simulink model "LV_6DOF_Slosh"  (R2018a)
settings: Solver=FixedStepAuto  StartTime=0.0  StopTime=489.8  FixedStep=0.0002  MaxStep=0.0001  RelTol=2e-6  EnableMultiTasking=on
InitFcn:
  | init
StopFcn:
  | pl
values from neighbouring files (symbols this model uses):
  accel = [97.3083,0,0]    [init.m]
  AcNoise = 0.1    [init.m]
  BBrcs = [82, 0.0, +3.375]    [init.m]
  Cdelay = 0.005    [init.m]
  Cza1 = FCS_Gains_Stg1(:, 5)    [init.m]
  d2r = pi/180    (= 0.0174532925199)    [init.m]    (also in pl.m; LQR_Design.m)
  Euler_0 = [90, 89.98, 0]*d2r    [init.m]
  fairing_mass = 1047.7*kg2slug    (= 71.7904994)    [init.m]
  Ie1 = 28.17    [init.m]
  Ie2 = 258.74    [init.m]
  Islosh = 1    [init.m]
  Isp = 65    [init.m]
  Ixxpr = Mass_Props(:,2)    [init.m]
  Ixypr = Mass_Props(:,5)    [init.m]
  Ixzpr = Mass_Props(:,6)    [init.m]
  Iyypr = Mass_Props(:,3)    [init.m]
  Iyzpr = Mass_Props(:,7)    [init.m]
  Izzpr = Mass_Props(:,4)    [init.m]
  Jdir = zeros(3,nt)    [init.m]
  JJ1 = Commands_2(:,2)    [init.m]
  JJ2 = Commands_2(:,3)    [init.m]
  JJ3 = Commands_2(:,4)    [init.m]
  Jloc = Jdir    [init.m]
  K_estim1 = FCS_Gains_Stg1(:,21)    [init.m]
  Kl_p1 = FCS_Gains_Stg1(:,12)    [init.m]
  Kl_phi1 = FCS_Gains_Stg1(:,11)    [init.m]
  Km_alfa1 = FCS_Gains_Stg1(:, 8)    [init.m]
  Km_alfin = FCS_Gains_Stg1(:,10)    [init.m]
  Km_q1 = FCS_Gains_Stg1(:, 7)    [init.m]
  Km_q2 = FCS_Gains_Stg2(:,5)    [init.m]
  Km_thet1 = FCS_Gains_Stg1(:, 6)    [init.m]
  Km_thet2 = FCS_Gains_Stg2(:,4)    [init.m]
  Km_thin1 = FCS_Gains_Stg1(:, 9)    [init.m]
  Km_thin2 = FCS_Gains_Stg2(:,6)    [init.m]
  Kmix2 = [ 0,   -1,    0;          0,    0,   -1]    [init.m]
  Kml1_1 = ee*FCS_Gains_Stg1(:,18)    [init.m]
  Kml2_1 = ee*FCS_Gains_Stg1(:,19)    [init.m]
  Kml2_2 = ee*FCS_Gains_Stg2(:,10)    [init.m]
  Kn_beta1 = FCS_Gains_Stg1(:,15)    [init.m]
  Kn_betin = FCS_Gains_Stg1(:,17)    [init.m]
  Kn_psi1 = FCS_Gains_Stg1(:,13)    [init.m]
  Kn_psi2 = FCS_Gains_Stg2(:,7)    [init.m]
  Kn_psin1 = FCS_Gains_Stg1(:,16)    [init.m]
  Kn_psin2 = FCS_Gains_Stg2(:,9)    [init.m]
  Kn_r1 = FCS_Gains_Stg1(:,14)    [init.m]
  Kn_r2 = FCS_Gains_Stg2(:,8)    [init.m]
  Le1 = 1.203    [init.m]
  Le2 = 2.892    [init.m]
  Massgn1 = ee*FCS_Gains_Stg1(:,2)    [init.m]
  Massgn2 = ee*FCS_Gains_Stg2(:,2)    [init.m]
  mdot1 = 2.5058    [init.m]
  mdot2 = 2.5058    [init.m]
  me1 = 9.325    [init.m]
  me2 = 13.927    [init.m]
  mrc = [x_ref, y_ref, z_ref]    [init.m]
  Msfue = Slosh(:,3)    [init.m]
  Mslox = Slosh(:,2)    [init.m]
  msspr = Mass_Props(:,1)    [init.m]
  Mvsls = Slosh(:,1)    [init.m]
  post_sep_wait = 4    [init.m]
  pre_sep_wait = 4    [init.m]
  Qbar1 = FCS_Gains_Stg1(:, 4)    [init.m]
  qtc1 = interp1(timi2(1:iend),Commands_2(1:iend, 9),timi2,'linear','extrap')    [init.m]
  qtc2 = interp1(timi2(1:iend),Commands_2(1:iend,10),timi2,'linear','extrap')    [init.m]
  qtc3 = interp1(timi2(1:iend),Commands_2(1:iend,11),timi2,'linear','extrap')    [init.m]
  qtc4 = interp1(timi2(1:iend),Commands_2(1:iend,12),timi2,'linear','extrap')    [init.m]
  r2d = 1/d2r    (= 57.2957795131)    [init.m]    (also in pl.m; LQR_Design.m)
  RBrcs = [82, +3.375, 0.0]    [init.m]
  Rfuel = Slosh(:,11)    [init.m]
  Rlox = Slosh(:,10)    [init.m]
  s1_dry_mass = 445.4969    [init.m]
  s1_init_prop_mass = 3.8002e+03    (= 3800.2)    [init.m]
  s2_dry_mass = 175.9451    [init.m]
  s2_init_prop_mass = 801.7606    [init.m]
  sp = 7.52    [init.m]
  Sref = 44.4146    [init.m]
  stage_to_fairing_sep_time = 34.7    [init.m]
  T3b = 176.6    [init.m]
  TBrcs = [82, 0.0, -3.375]    [init.m]
  thpnd = 15    [init.m]
  timi2 = Commands_2(:,1)    [init.m]
  TqLoad = 1    [init.m]
  tvc10 = [Xgmb2, 0.0,  0.0]    [init.m]
  tvc2 = [Xgmb1,  1.0202,  -2.4638]    [init.m]
  tvc3 = [Xgmb1, -1.0202,  -2.4638]    [init.m]
  tvc4 = [Xgmb1, -2.4638,  -1.0202]    [init.m]
  tvc5 = [Xgmb1, -2.4638,   1.0202]    [init.m]
  tvc6 = [Xgmb1, -1.0202,   2.4638]    [init.m]
  tvc7 = [Xgmb1,  1.0202,   2.4638]    [init.m]
  tvc8 = [Xgmb1,  2.4638,   1.0202]    [init.m]
  tvc9 = [Xgmb1,  0.0,      0.0]    [init.m]
  velpnd = 3    [init.m]
  Vrelgn1 = FCS_Gains_Stg1(:, 3)    [init.m]
  Vrelgn2 = FCS_Gains_Stg2(:,3)    [init.m]
  W_lowp1 = FCS_Gains_Stg1(:,22)    [init.m]
  W_nfilt1 = FCS_Gains_Stg1(:,20)    [init.m]
  Xcgpr = Mass_Props(:,8)    [init.m]
  Xfuel = Slosh(:,9)    [init.m]
  Xgmb1 = 10.7062    [init.m]
  Xgmb2 = 82.538    [init.m]
  Xlox = Slosh(:,8)    [init.m]
  Ycgpr = Mass_Props(:,9)    [init.m]
  Zcgpr = Mass_Props(:,10)    [init.m]
  Ztfue = Slosh(:,7)    [init.m]
  Ztlox = Slosh(:,6)    [init.m]
undefined symbols (not defined in the file or in its folder): Cl, Cl2, Cm, Cm2, Cn, Cn2, Continuous, cosd, CX, CX2, CY, CY2, CZ, CZ2, Dryden, Earth, F, ft, Isp1, Isp2, km, Kmix1, LBrcs, Light, MIL, q, r, sigbuilder_block, sind, STD, tvc1, WGS84
libraries: sharedutil x28, Actuator_Lib x18, simulink x4, aerolibasang x3, aerolibwind2 x3, sharedtransform x3, aerolibobsolete x2, aerolibconvert2 x2, aerolibatmos2 x1, aerolibadyn x1, aerolibutil x1
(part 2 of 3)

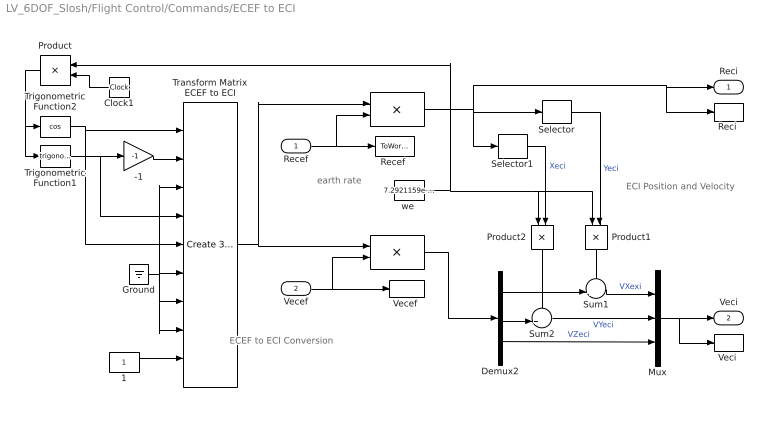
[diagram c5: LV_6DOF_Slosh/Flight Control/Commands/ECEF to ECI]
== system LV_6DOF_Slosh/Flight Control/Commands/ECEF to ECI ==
  note: ECI Position and Velocity
  note: ECEF to ECI Conversion
  note: earth rate
  Recef : Inport
  Vecef : Inport  Port=2
  " " : Product  Multiplication=Matrix(*)
  "  " : Product  Multiplication=Matrix(*)
  -1 : Gain  Gain=-1
  1 : Constant
  Clock1 : Clock
  Demux2 : Demux  Outputs=3
  Ground : Ground
  Mux : Mux  Inputs=3
  Product : Product
  Product1 : Product
  Product2 : Product
  "Recef " : ToWorkspace  VariableName=Recef  SampleTime=-1
  "Reci " : ToWorkspace  VariableName=Reci  SampleTime=-1
  Selector : Selector  InputPortWidth=3  IndexOptions=Index vector (dialog)  Indices=[2]  OutputSizes=1
  Selector1 : Selector  InputPortWidth=3  IndexOptions=Index vector (dialog)  Indices=[1]  OutputSizes=1
  Sum1 : Sum  Inputs=-+|
  Sum2 : Sum  Inputs=++|
  Transform Matrix ECEF to ECI : sharedutil/Create 3x3 Matrix  aMode=aMode
  Trigonometric Function1 : Trigonometry
  Trigonometric Function2 : Trigonometry  Operator=cos
  "Vecef " : ToWorkspace  VariableName=Vecef  SampleTime=-1
  "Veci " : ToWorkspace  VariableName=Veci  SampleTime=-1
  "we " : Constant  Value=7.2921159e-5
  Reci : Outport
  Veci : Outport  Port=2
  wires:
  Product/1 -> Trigonometric Function1/1, Trigonometric Function2/1
  Trigonometric Function2/1 -> Transform Matrix ECEF to ECI/5, Transform Matrix ECEF to ECI/1
  -1/1 -> Transform Matrix ECEF to ECI/2
  Trigonometric Function1/1 -> Transform Matrix ECEF to ECI/4, -1/1
  1/1 -> Transform Matrix ECEF to ECI/9
  Ground/1 -> Transform Matrix ECEF to ECI/3, Transform Matrix ECEF to ECI/7, Transform Matrix ECEF to ECI/8, Transform Matrix ECEF to ECI/6
  Transform Matrix ECEF to ECI/1 -> " "/1, "  "/1
  " "/1 -> Selector1/1, Selector/1, "Reci "/1, Reci/1
  Demux2/3 -> Mux/3  "VZeci"
  Sum1/1 -> Mux/1  "VXexi"
  Demux2/1 -> Sum1/2
  Sum2/1 -> Mux/2  "VYeci"
  Demux2/2 -> Sum2/2
  "  "/1 -> Demux2/1
  Product1/1 -> Sum1/1
  Product2/1 -> Sum2/1
  Selector/1 -> Product1/2  "Yeci"
  Selector1/1 -> Product2/2  "Xeci"
  "we "/1 -> Product/1, Product2/1, Product1/1
  Mux/1 -> "Veci "/1, Veci/1
  Clock1/1 -> Product/2
  Recef/1 -> " "/2, "Recef "/1
  Vecef/1 -> "  "/2, "Vecef "/1

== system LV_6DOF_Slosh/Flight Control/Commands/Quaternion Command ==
  1-D Lookup Table : Lookup_n-D  NumberOfTableDimensions=1  BreakpointsForDimension1=timi2  Table=qtc1  InternalRulePriority=Speed  RndMeth=Simplest
  1-D Lookup Table1 : Lookup_n-D  NumberOfTableDimensions=1  BreakpointsForDimension1=timi2  Table=qtc2  InternalRulePriority=Speed  RndMeth=Simplest
  1-D Lookup Table2 : Lookup_n-D  NumberOfTableDimensions=1  BreakpointsForDimension1=timi2  Table=qtc3  InternalRulePriority=Speed  RndMeth=Simplest
  1-D Lookup Table3 : Lookup_n-D  NumberOfTableDimensions=1  BreakpointsForDimension1=timi2  Table=qtc4  InternalRulePriority=Speed  RndMeth=Simplest
  Clock : Clock
  Mux1 : Mux
  Quatin : Outport
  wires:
  Clock/1 -> 1-D Lookup Table/1, 1-D Lookup Table1/1, 1-D Lookup Table2/1, 1-D Lookup Table3/1
  1-D Lookup Table3/1 -> Mux1/4
  1-D Lookup Table2/1 -> Mux1/3
  1-D Lookup Table/1 -> Mux1/1
  1-D Lookup Table1/1 -> Mux1/2
  Mux1/1 -> Quatin/1

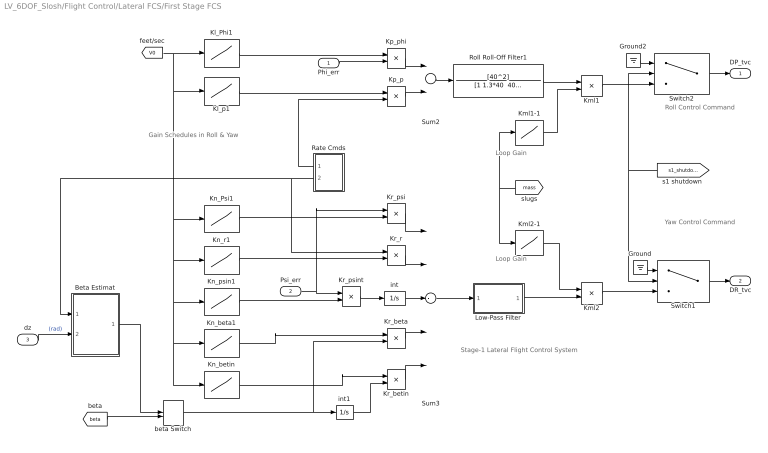
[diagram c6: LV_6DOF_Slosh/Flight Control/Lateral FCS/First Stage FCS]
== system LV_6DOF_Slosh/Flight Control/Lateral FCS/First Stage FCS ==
  note: Gain Schedules in Roll & Yaw
  note: Stage-1 Lateral Flight Control System
  note: Roll Control Command
  note: Yaw Control Command
  note: Loop Gain
  note: Loop Gain
  Phi_err : Inport
  Psi_err : Inport  Port=2
  dz : Inport  Port=3
  Beta Estimat : Subsystem
  Ground : Ground
  Ground2 : Ground
  Kl_Phi1 : Lookup  InputValues=Vrelgn1  Table=Kl_phi1
  Kl_p1 : Lookup  InputValues=Vrelgn1  Table=Kl_p1
  Kml1 : Product
  Kml1-1 : Lookup  InputValues=Massgn1  Table=Kml1_1
  Kml2 : Product
  Kml2-1 : Lookup  InputValues=Massgn1  Table=Kml2_1
  Kn_Psi1 : Lookup  InputValues=Vrelgn1  Table=Kn_psi1
  Kn_beta1 : Lookup  InputValues=Vrelgn1  Table=Kn_beta1
  Kn_betin : Lookup  InputValues=Vrelgn1  Table=Kn_betin
  Kn_psin1 : Lookup  InputValues=Vrelgn1  Table=Kn_psin1
  Kn_r1 : Lookup  InputValues=Vrelgn1  Table=Kn_r1
  Kp_p : Product
  Kp_phi : Product
  Kr_beta : Product
  Kr_betin : Product
  Kr_psi : Product
  Kr_psint : Product
  Kr_r : Product
  Low-Pass Filter : Subsystem
  Rate Cmds : Subsystem
  Roll Roll-Off Filter1 : TransferFcn  Numerator=[40^2]  Denominator="[1 1.3*40  40^2]"
  Sum2 : Sum  Inputs=--
  Sum3 : Sum  Inputs=-----
  Switch1 : Switch  Criteria=u2 > Threshold
  Switch2 : Switch  Criteria=u2 > Threshold
  beta Switch : ManualSwitch
  int : Integrator
  int1 : Integrator
  DP_tvc : Outport
  DR_tvc : Outport  Port=2
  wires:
  Psi_err/1 -> Kr_psint/1, Kr_psi/1
  [mass] -> Kml1-1/1, Kml2-1/1
  [V0] -> Kn_betin/1, Kn_beta1/1, Kn_psin1/1, Kn_r1/1, Kn_Psi1/1, Kl_p1/1, Kl_Phi1/1
  beta Switch/1 -> int1/1, Kr_beta/2
  Kp_p/1 -> Sum2/2
  Kml1-1/1 -> Kml1/2
  Kp_phi/1 -> Sum2/1
  Switch2/1 -> DP_tvc/1
  Ground2/1 -> Switch2/1
  Kml2-1/1 -> Kml2/1
  Kml1/1 -> Switch2/3
  Sum2/1 -> Roll Roll-Off Filter1/1
  Kml2/1 -> Switch1/3
  Ground/1 -> Switch1/1
  [s1_shutdown] -> Switch2/2, Switch1/2
  Switch1/1 -> DR_tvc/1
  Kr_psi/1 -> Sum3/1
  Kr_r/1 -> Sum3/2
  Kr_betin/1 -> Sum3/5
  Kr_psint/1 -> int/1
  Kr_beta/1 -> Sum3/4
  Phi_err/1 -> Kp_phi/2
  dz/1 -> Beta Estimat/2(dz)  "(rad)"
  [beta] -> beta Switch/2
  Beta Estimat/1(betest) -> beta Switch/1
  int1/1 -> Kr_betin/2
  Roll Roll-Off Filter1/1 -> Kml1/1
  Rate Cmds/2(Rcm) -> Kr_r/1, Beta Estimat/1(r)
  Rate Cmds/1(Pcm) -> Kp_p/2
  Kl_p1/1 -> Kp_p/1
  Kl_Phi1/1 -> Kp_phi/1
  Sum3/1 -> Low-Pass Filter/1(u)
  Low-Pass Filter/1(y) -> Kml2/2
  int/1 -> Sum3/3
  Kn_Psi1/1 -> Kr_psi/2
  Kn_r1/1 -> Kr_r/2
  Kn_psin1/1 -> Kr_psint/2
  Kn_beta1/1 -> Kr_beta/1
  Kn_betin/1 -> Kr_betin/1

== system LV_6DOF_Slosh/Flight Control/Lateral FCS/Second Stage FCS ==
  note: Yaw Gain Schedules
  note: Stage-2 Lateral Flight Control System
  note: Yaw Control Command
  note: Loop Gain
  Psi_err : Inport
  Ground1 : Ground
  Integr : Subsystem
  Kml2-2 : Lookup  InputValues=Massgn2  Table=Kml2_2
  Kml2_2 : Product
  Kn_Psi2 : Lookup  InputValues=Vrelgn2  Table=Kn_psi2
  Kn_psin2 : Lookup  InputValues=Vrelgn2  Table=Kn_psin2
  Kn_r2 : Lookup  InputValues=Vrelgn2  Table=Kn_r2
  Kr_psi : Product
  Kr_psint : Product
  Kr_r : Product
  Select R : Selector  InputPortWidth=3  IndexOptions=Index vector (dialog)  Indices=[3]  OutputSizes=1
  Sum3 : Sum  Inputs=---
  Switch2 : Switch  Criteria=u2 > Threshold
  DR_tvc : Outport
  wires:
  [mass] -> Kml2-2/1
  [V0] -> Kn_Psi2/1, Kn_r2/1, Kn_psin2/1
  Psi_err/1 -> Integr/1(in), Kr_psi/1
  Sum3/1 -> Kml2_2/2
  Kml2-2/1 -> Kml2_2/1
  Select R/1 -> Kr_r/1
  [Gyros] -> Select R/1
  Ground1/1 -> Switch2/3
  Kml2_2/1 -> Switch2/1
  [s2_startup] -> Switch2/2
  Switch2/1 -> DR_tvc/1
  Kr_psi/1 -> Sum3/1
  Kr_r/1 -> Sum3/2
  Kr_psint/1 -> Sum3/3
  Kn_Psi2/1 -> Kr_psi/2
  Kn_r2/1 -> Kr_r/2
  Kn_psin2/1 -> Kr_psint/2
  Integr/1(ou) -> Kr_psint/1

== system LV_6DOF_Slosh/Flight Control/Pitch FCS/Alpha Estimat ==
  note: Qbar*Sref*Cza*alfa
  note: Alpha Estimator
  dy : Inport
  q : Inport  Port=2
  1/9 : Gain  Gain=1/9
  3 : Gain  Gain=15
  Czalfa : Lookup  InputValues=Vrelgn1  Table=Cza1
  Demux : Demux  Outputs=8
  Mass : Product
  Nz Washout : TransferFcn  Numerator="[1  0]"  Denominator="[0.015  1]"
  Product : Product  Inputs=4
  Qbar : Lookup  InputValues=Vrelgn1  Table=Qbar1
  Selector : Selector  InputPortWidth=3  IndexOptions=Index vector (dialog)  Indices=[3]  OutputSizes=1
  Selector1 : Selector  InputPortWidth=2  IndexOptions=Index vector (dialog)  Indices=[1]  OutputSizes=1
  Slosh-Notch : Subsystem
  Sref : Constant  Value=Sref
  Sum : Sum  Inputs=++|
  Sum of Elements : Sum  Inputs=++++++++
  Sum2 : Sum  Inputs=---
  Thrust*dy : Product
  d2r : Gain  Gain=d2r
  alfest : Outport
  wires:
  Slosh-Notch/1(Out) -> Product/1, d2r/1  "alfa (deg)"
  3/1 -> Sum/1
  Sum2/1 -> Slosh-Notch/1(In)
  Product/1 -> Sum2/3
  Mass/1 -> Sum2/1
  d2r/1 -> alfest/1
  Sum/1 -> Mass/2
  [mass] -> Mass/1
  Thrust*dy/1 -> Sum2/2  "Fz"
  [V0] -> Qbar/1, Czalfa/1
  Qbar/1 -> Product/4
  Sref/1 -> Product/2
  Czalfa/1 -> Product/3
  [Axlrm] -> Selector/1  "(ft/sec^2)"
  Selector/1 -> Sum/2  "Zdd"
  [Teng] -> Selector1/1  "(lbf)"
  Demux/8 -> Sum of Elements/8
  Demux/6 -> Sum of Elements/6
  dy/1 -> Demux/1  "(rad)"
  Sum of Elements/1 -> Thrust*dy/2
  Selector1/1 -> 1/9/1
  Demux/4 -> Sum of Elements/4
  1/9/1 -> Thrust*dy/1
  Demux/5 -> Sum of Elements/5
  Demux/3 -> Sum of Elements/3
  Demux/7 -> Sum of Elements/7
  Demux/2 -> Sum of Elements/2
  Demux/1 -> Sum of Elements/1
  Nz Washout/1 -> 3/1
  q/1 -> Nz Washout/1

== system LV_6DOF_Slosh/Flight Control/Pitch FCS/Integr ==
  in : Inport
  Ground2 : Ground
  Switch : Switch  Criteria=u2 > Threshold
  int3 : Integrator
  ou : Outport
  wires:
  Ground2/1 -> Switch/3
  [s2_startup] -> Switch/2
  Switch/1 -> int3/1
  in/1 -> Switch/1
  int3/1 -> ou/1

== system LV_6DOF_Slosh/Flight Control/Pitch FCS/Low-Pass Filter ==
  note: Variable Low Pass Filter
  note: Filter Bandwidth varies with Rel. Velocity
  u : Inport
  2.zeta.w : Subsystem
  Sum2 : Sum  Inputs=|+-
  Sum3 : Sum  Inputs=-+|
  W_lowp1 : Lookup  InputValues=Vrelgn1  Table=W_lowp1
  int1 : Integrator
  int2 : Integrator
  "w^2 " : Subsystem
  y : Outport
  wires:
  [V0] -> W_lowp1/1
  Sum3/1 -> "w^2 "/1(in)
  int1/1 -> 2.zeta.w/1(in), int2/1
  Sum2/1 -> int1/1
  "w^2 "/1(ou) -> Sum2/1
  2.zeta.w/1(ou) -> Sum2/2
  int2/1 -> Sum3/1, y/1
  u/1 -> Sum3/2
  W_lowp1/1 -> [Wlp]

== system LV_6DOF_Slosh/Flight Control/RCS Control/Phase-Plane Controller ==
  note: Number of Selected Jets
  note: Phase-Plane / Jet-Select Logic
  note: Rotation Vector
  note: Jet Forces
  note: Attitude and Rate Errors
  note: RCS Locations and Directions
  rater : Inport
  atter : Inport  Port=2
  "  eu" : ToWorkspace  VariableName=eu  SampleTime=-1
  Constant : Constant  Value=Jloc
  Constant1 : Constant  Value=Jdir
  Isel : Scope
  MATLAB Function : MATLAB Function  TreatAsAtomicUnit=on
  Xcg : Selector  InputPortWidth=3  IndexOptions=Index vector (dialog)  Indices=[1]  OutputSizes=1
  f(i) : Outport
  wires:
  Xcg/1 -> MATLAB Function/6(Xcg)
  [CG] -> Xcg/1
  MATLAB Function/1(fp) -> f(i)/1
  [Izz] -> MATLAB Function/5(J33)
  [Iyy] -> MATLAB Function/4(J22)
  [Ixx] -> MATLAB Function/3(J11)
  MATLAB Function/2(eu) -> "  eu"/1
  rater/1 -> MATLAB Function/1(Rater)
  atter/1 -> MATLAB Function/2(Atter)
  MATLAB Function/3(Isel) -> Isel/1
  Constant/1 -> MATLAB Function/8(Jloc)
  Constant1/1 -> MATLAB Function/7(Jdir)

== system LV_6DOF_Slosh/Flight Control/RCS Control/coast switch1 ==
  in : Inport
  Ground1 : Ground
  Logical Operator : Logic  Operator=NAND  AllPortsSameDT=off  OutDataTypeStr=boolean
  Switch1 : Switch  Criteria=u2 > Threshold
  ou : Outport
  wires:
  Logical Operator/1 -> Switch1/2
  [s2_startup] -> Logical Operator/2
  [stage_sep] -> Logical Operator/1
  in/1 -> Switch1/1
  Ground1/1 -> Switch1/3
  Switch1/1 -> ou/1

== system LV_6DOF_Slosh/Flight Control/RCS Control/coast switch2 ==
  in : Inport
  Ground1 : Ground
  Logical Operator : Logic  Operator=NAND  AllPortsSameDT=off  OutDataTypeStr=boolean
  Switch1 : Switch  Criteria=u2 > Threshold
  ou : Outport
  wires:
  Logical Operator/1 -> Switch1/2
  [s2_startup] -> Logical Operator/2
  [stage_sep] -> Logical Operator/1
  in/1 -> Switch1/1
  Ground1/1 -> Switch1/3
  Switch1/1 -> ou/1

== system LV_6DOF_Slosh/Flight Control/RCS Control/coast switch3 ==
  in : Inport
  Ground1 : Ground
  Logical Operator : Logic  Operator=NAND  AllPortsSameDT=off  OutDataTypeStr=boolean
  Switch1 : Switch  Criteria=u2 > Threshold
  ou : Outport
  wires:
  Logical Operator/1 -> Switch1/2
  [s2_startup] -> Logical Operator/2
  [stage_sep] -> Logical Operator/1
  in/1 -> Switch1/1
  Ground1/1 -> Switch1/3
  Switch1/1 -> ou/1

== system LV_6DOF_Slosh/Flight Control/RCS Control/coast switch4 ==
  in : Inport
  Ground1 : Ground
  Logical Operator : Logic  Operator=NAND  AllPortsSameDT=off  OutDataTypeStr=boolean
  Switch1 : Switch  Criteria=u2 > Threshold
  ou : Outport
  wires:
  Logical Operator/1 -> Switch1/2
  [s2_startup] -> Logical Operator/2
  [stage_sep] -> Logical Operator/1
  in/1 -> Switch1/1
  Ground1/1 -> Switch1/3
  Switch1/1 -> ou/1

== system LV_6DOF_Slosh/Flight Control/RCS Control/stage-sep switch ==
  in : Inport
  Ground1 : Ground
  Switch1 : Switch  Criteria=u2 > Threshold
  ou : Outport
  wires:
  in/1 -> Switch1/1
  Ground1/1 -> Switch1/3
  Switch1/1 -> ou/1
  [stage_sep] -> Switch1/2

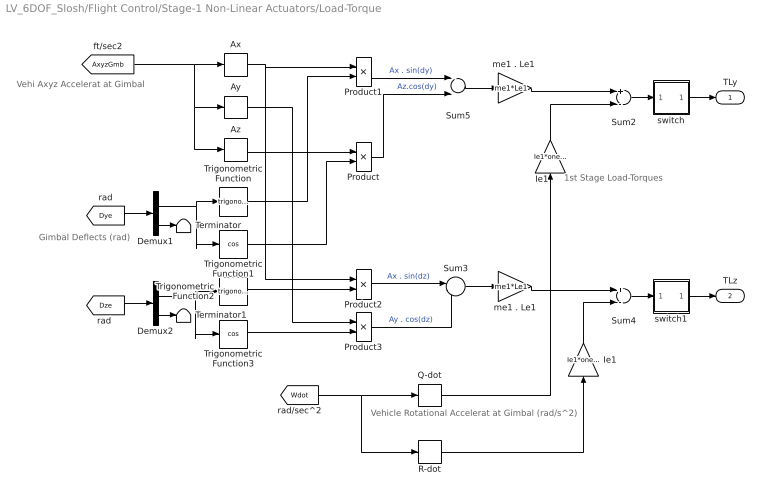
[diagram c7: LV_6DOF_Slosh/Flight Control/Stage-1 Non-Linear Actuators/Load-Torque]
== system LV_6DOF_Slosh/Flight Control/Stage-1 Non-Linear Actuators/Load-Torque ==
  note: Vehi Axyz Accelerat at Gimbal
  note: 1st Stage Load-Torques
  note: Gimbal Deflects (rad)
  note: Vehicle Rotational Accelerat at Gimbal (rad/s^2)
  Ax : Selector  InputPortWidth=3  IndexOptions=Index vector (dialog)  Indices=[1]  OutputSizes=1
  Ay : Selector  InputPortWidth=3  IndexOptions=Index vector (dialog)  Indices=[2]  OutputSizes=1
  Az : Selector  InputPortWidth=3  IndexOptions=Index vector (dialog)  Indices=[3]  OutputSizes=1
  Demux1 : Demux  Outputs=[8,1]
  Demux2 : Demux  Outputs=[8,1]
  Ie1 : Gain  Gain=Ie1*ones(8,1)  Multiplication=Matrix(K*u)
  "Ie1 " : Gain  Gain=Ie1*ones(8,1)  Multiplication=Matrix(K*u)
  Product{,1..3} (4 alike) : Product
  Q-dot : Selector  InputPortWidth=3  IndexOptions=Index vector (dialog)  Indices=[2]  OutputSizes=1
  R-dot : Selector  InputPortWidth=3  IndexOptions=Index vector (dialog)  Indices=[3]  OutputSizes=1
  Sum2 : Sum  Inputs=+-
  Sum3 : Sum  Inputs=|-+
  Sum4 : Sum  Inputs=+-
  Sum5 : Sum  Inputs=--
  Terminator : Terminator
  Terminator1 : Terminator
  Trigonometric Function : Trigonometry
  Trigonometric Function1 : Trigonometry  Operator=cos
  Trigonometric Function2 : Trigonometry
  Trigonometric Function3 : Trigonometry  Operator=cos
  me1 . Le1 : Gain  Gain=me1*Le1
  "me1 . Le1 " : Gain  Gain=me1*Le1
  switch : Subsystem
  switch1 : Subsystem
  TLy : Outport
  TLz : Outport  Port=2
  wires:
  [Wdot] -> R-dot/1, Q-dot/1
  Q-dot/1 -> Ie1/1
  R-dot/1 -> "Ie1 "/1
  [AxyzGmb] -> Ay/1, Az/1, Ax/1
  [Dye] -> Demux1/1
  Demux1/2 -> Terminator/1
  Demux1/1 -> Trigonometric Function1/1, Trigonometric Function/1
  Az/1 -> Product/1
  Trigonometric Function1/1 -> Product/2
  Product/1 -> Sum5/2  "Az.cos(dy)"
  Ax/1 -> Product2/1, Product1/1
  Trigonometric Function/1 -> Product1/2
  Product1/1 -> Sum5/1  "Ax . sin(dy)"
  Ie1/1 -> Sum2/2
  Sum2/1 -> switch/1(in)
  [Dze] -> Demux2/1
  Demux2/1 -> Trigonometric Function3/1, Trigonometric Function2/1
  Demux2/2 -> Terminator1/1
  Trigonometric Function2/1 -> Product2/2
  Product2/1 -> Sum3/1  "Ax . sin(dz)"
  Trigonometric Function3/1 -> Product3/2
  Ay/1 -> Product3/1
  Product3/1 -> Sum3/2  "Ay . cos(dz)"
  Sum3/1 -> me1 . Le1/1
  Sum5/1 -> "me1 . Le1 "/1
  "me1 . Le1 "/1 -> Sum2/1
  me1 . Le1/1 -> Sum4/1
  "Ie1 "/1 -> Sum4/2
  switch/1(ou) -> TLy/1
  Sum4/1 -> switch1/1(in)
  switch1/1(ou) -> TLz/1

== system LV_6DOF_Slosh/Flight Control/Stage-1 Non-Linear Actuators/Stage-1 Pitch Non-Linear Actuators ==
  Dy_cmd : Inport
  Ty_Load : Inport  Port=2
  Add : Sum  Inputs=8
  Demux1 : Demux  Outputs=8
  Demux2 : Demux  Outputs=8
  Demux3 : Demux  Outputs=8
  Mux1 : Mux  Inputs=8
  Mux2 : Mux  Inputs=8
  Mux5 : Mux  Inputs=8
  NonLinear Actuator{,1..6,8} (8 alike) : Actuator_Lib/Stage1 Actuator
  RT : RateTransition  OutPortSampleTime=0.0002
  Shaft Position Noise 0.1 deg : UniformRandomNumber  Minimum=-[1 1 1 1 1 1 1 1]*AcNoise*d2r  Maximum=[1 1 1 1 1 1 1 1]*AcNoise*d2r  Seed=[10,15,20,25,30,35,40,45]  SampleTime=0.01
  Dy_out : Outport
  Dy_pow : Outport  Port=2
  Dy_dd : Outport  Port=3
  Xpy : Outport  Port=4
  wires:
  NonLinear Actuator8/1 -> Mux5/8
  NonLinear Actuator6/1 -> Mux5/7
  NonLinear Actuator5/1 -> Mux5/6
  NonLinear Actuator4/1 -> Mux5/5
  NonLinear Actuator3/1 -> Mux5/4
  NonLinear Actuator2/1 -> Mux5/3
  NonLinear Actuator1/1 -> Mux5/2
  NonLinear Actuator/1 -> Mux5/1
  Demux1/7 -> NonLinear Actuator6/1
  Demux1/6 -> NonLinear Actuator5/1
  Demux1/5 -> NonLinear Actuator4/1
  Demux1/4 -> NonLinear Actuator3/1
  Demux1/3 -> NonLinear Actuator2/1
  Demux1/2 -> NonLinear Actuator1/1
  Demux1/8 -> NonLinear Actuator8/1
  Demux1/1 -> NonLinear Actuator/1
  Mux5/1 -> Dy_out/1
  Dy_cmd/1 -> Demux1/1
  Demux2/8 -> NonLinear Actuator8/2
  Demux2/7 -> NonLinear Actuator6/2
  Demux2/6 -> NonLinear Actuator5/2
  Demux2/5 -> NonLinear Actuator4/2
  Demux2/4 -> NonLinear Actuator3/2
  Demux2/3 -> NonLinear Actuator2/2
  Demux2/2 -> NonLinear Actuator1/2
  Demux2/1 -> NonLinear Actuator/2
  RT/1 -> Demux2/1
  NonLinear Actuator/2 -> Add/1
  NonLinear Actuator1/2 -> Add/2
  NonLinear Actuator2/2 -> Add/3
  NonLinear Actuator3/2 -> Add/4
  NonLinear Actuator4/2 -> Add/5
  NonLinear Actuator5/2 -> Add/6
  NonLinear Actuator6/2 -> Add/7
  NonLinear Actuator8/2 -> Add/8
  Add/1 -> Dy_pow/1
  NonLinear Actuator/3 -> Mux1/1
  NonLinear Actuator1/3 -> Mux1/2
  NonLinear Actuator2/3 -> Mux1/3
  NonLinear Actuator3/3 -> Mux1/4
  NonLinear Actuator4/3 -> Mux1/5
  NonLinear Actuator5/3 -> Mux1/6
  NonLinear Actuator6/3 -> Mux1/7
  NonLinear Actuator8/3 -> Mux1/8
  Mux1/1 -> Dy_dd/1
  Shaft Position Noise 0.1 deg/1 -> RT/1
  NonLinear Actuator/4 -> Mux2/1
  NonLinear Actuator1/4 -> Mux2/2
  NonLinear Actuator2/4 -> Mux2/3
  NonLinear Actuator3/4 -> Mux2/4
  NonLinear Actuator4/4 -> Mux2/5
  NonLinear Actuator5/4 -> Mux2/6
  NonLinear Actuator6/4 -> Mux2/7
  NonLinear Actuator8/4 -> Mux2/8
  Mux2/1 -> Xpy/1
  Demux3/1 -> NonLinear Actuator/3
  Demux3/2 -> NonLinear Actuator1/3
  Demux3/3 -> NonLinear Actuator2/3
  Demux3/4 -> NonLinear Actuator3/3
  Demux3/5 -> NonLinear Actuator4/3
  Demux3/6 -> NonLinear Actuator5/3
  Demux3/7 -> NonLinear Actuator6/3
  Demux3/8 -> NonLinear Actuator8/3
  Ty_Load/1 -> Demux3/1

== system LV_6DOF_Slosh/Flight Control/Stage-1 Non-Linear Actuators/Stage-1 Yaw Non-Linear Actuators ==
  Dz_cmd : Inport
  Tz_Load : Inport  Port=2
  Add : Sum  Inputs=8
  Demux1 : Demux  Outputs=8
  Demux2 : Demux  Outputs=8
  Demux3 : Demux  Outputs=8
  Mux1 : Mux  Inputs=8
  Mux2 : Mux  Inputs=8
  Mux5 : Mux  Inputs=8
  NonLinear Actuator{,1..6,8} (8 alike) : Actuator_Lib/Stage1 Actuator
  RT : RateTransition  OutPortSampleTime=0.0002
  Shaft Position Noise 0.1 deg : UniformRandomNumber  Minimum=-[1 1 1 1 1 1 1 1]*AcNoise*d2r  Maximum=[1 1 1 1 1 1 1 1]*AcNoise*d2r  Seed=[10,15,20,25,30,35,40,45]  SampleTime=0.01
  Dz_out : Outport
  Dz_pow : Outport  Port=2
  Dz_dd : Outport  Port=3
  Xpz : Outport  Port=4
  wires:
  NonLinear Actuator8/1 -> Mux5/8
  NonLinear Actuator6/1 -> Mux5/7
  NonLinear Actuator5/1 -> Mux5/6
  NonLinear Actuator4/1 -> Mux5/5
  NonLinear Actuator3/1 -> Mux5/4
  NonLinear Actuator2/1 -> Mux5/3
  NonLinear Actuator1/1 -> Mux5/2
  NonLinear Actuator/1 -> Mux5/1
  Demux1/7 -> NonLinear Actuator6/1
  Demux1/6 -> NonLinear Actuator5/1
  Demux1/5 -> NonLinear Actuator4/1
  Demux1/4 -> NonLinear Actuator3/1
  Demux1/3 -> NonLinear Actuator2/1
  Demux1/2 -> NonLinear Actuator1/1
  Demux1/8 -> NonLinear Actuator8/1
  Demux1/1 -> NonLinear Actuator/1
  Mux5/1 -> Dz_out/1
  Dz_cmd/1 -> Demux1/1
  Demux2/8 -> NonLinear Actuator8/2
  Demux2/7 -> NonLinear Actuator6/2
  Demux2/6 -> NonLinear Actuator5/2
  Demux2/5 -> NonLinear Actuator4/2
  Demux2/4 -> NonLinear Actuator3/2
  Demux2/3 -> NonLinear Actuator2/2
  Demux2/2 -> NonLinear Actuator1/2
  Demux2/1 -> NonLinear Actuator/2
  RT/1 -> Demux2/1
  NonLinear Actuator/2 -> Add/1
  NonLinear Actuator1/2 -> Add/2
  NonLinear Actuator2/2 -> Add/3
  NonLinear Actuator3/2 -> Add/4
  NonLinear Actuator4/2 -> Add/5
  NonLinear Actuator5/2 -> Add/6
  NonLinear Actuator6/2 -> Add/7
  NonLinear Actuator8/2 -> Add/8
  Add/1 -> Dz_pow/1
  NonLinear Actuator/3 -> Mux1/1
  NonLinear Actuator1/3 -> Mux1/2
  NonLinear Actuator2/3 -> Mux1/3
  NonLinear Actuator3/3 -> Mux1/4
  NonLinear Actuator4/3 -> Mux1/5
  NonLinear Actuator5/3 -> Mux1/6
  NonLinear Actuator6/3 -> Mux1/7
  NonLinear Actuator8/3 -> Mux1/8
  Mux1/1 -> Dz_dd/1
  Shaft Position Noise 0.1 deg/1 -> RT/1
  NonLinear Actuator/4 -> Mux2/1
  NonLinear Actuator1/4 -> Mux2/2
  NonLinear Actuator2/4 -> Mux2/3
  NonLinear Actuator3/4 -> Mux2/4
  NonLinear Actuator4/4 -> Mux2/5
  NonLinear Actuator5/4 -> Mux2/6
  NonLinear Actuator6/4 -> Mux2/7
  NonLinear Actuator8/4 -> Mux2/8
  Mux2/1 -> Xpz/1
  Demux3/1 -> NonLinear Actuator/3
  Demux3/2 -> NonLinear Actuator1/3
  Demux3/3 -> NonLinear Actuator2/3
  Demux3/4 -> NonLinear Actuator3/3
  Demux3/5 -> NonLinear Actuator4/3
  Demux3/6 -> NonLinear Actuator5/3
  Demux3/7 -> NonLinear Actuator6/3
  Demux3/8 -> NonLinear Actuator8/3
  Tz_Load/1 -> Demux3/1

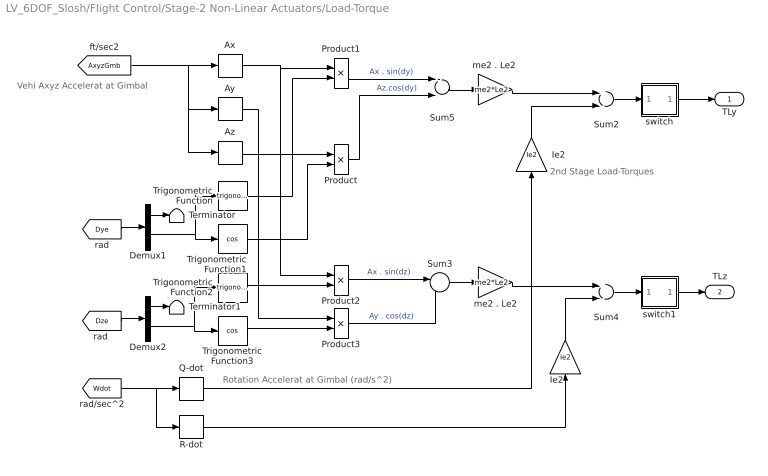
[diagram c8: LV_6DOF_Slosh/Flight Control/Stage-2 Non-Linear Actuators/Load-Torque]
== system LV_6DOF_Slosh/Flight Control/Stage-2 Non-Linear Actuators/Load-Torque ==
  note: Vehi Axyz Accelerat at Gimbal
  note: 2nd Stage Load-Torques
  note: Rotation Accelerat at Gimbal (rad/s^2)
  Ax : Selector  InputPortWidth=3  IndexOptions=Index vector (dialog)  Indices=[1]  OutputSizes=1
  Ay : Selector  InputPortWidth=3  IndexOptions=Index vector (dialog)  Indices=[2]  OutputSizes=1
  Az : Selector  InputPortWidth=3  IndexOptions=Index vector (dialog)  Indices=[3]  OutputSizes=1
  Demux1 : Demux  Outputs=[8,1]
  Demux2 : Demux  Outputs=[8,1]
  Ie2 : Gain  Gain=Ie2
  "Ie2 " : Gain  Gain=Ie2
  Product{,1..3} (4 alike) : Product
  Q-dot : Selector  InputPortWidth=3  IndexOptions=Index vector (dialog)  Indices=[2]  OutputSizes=1
  R-dot : Selector  InputPortWidth=3  IndexOptions=Index vector (dialog)  Indices=[3]  OutputSizes=1
  Sum2 : Sum  Inputs=+-
  Sum3 : Sum  Inputs=|-+
  Sum4 : Sum  Inputs=+-
  Sum5 : Sum  Inputs=--
  Terminator : Terminator
  Terminator1 : Terminator
  Trigonometric Function : Trigonometry
  Trigonometric Function1 : Trigonometry  Operator=cos
  Trigonometric Function2 : Trigonometry
  Trigonometric Function3 : Trigonometry  Operator=cos
  me2 . Le2 : Gain  Gain=me2*Le2
  "me2 . Le2 " : Gain  Gain=me2*Le2
  switch : Subsystem
  switch1 : Subsystem
  TLy : Outport
  TLz : Outport  Port=2
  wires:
  [Wdot] -> R-dot/1, Q-dot/1
  Q-dot/1 -> "Ie2 "/1
  [AxyzGmb] -> Ay/1, Az/1, Ax/1
  [Dze] -> Demux2/1
  [Dye] -> Demux1/1
  Demux1/2 -> Trigonometric Function/1, Trigonometric Function1/1
  Demux2/2 -> Trigonometric Function2/1, Trigonometric Function3/1
  Demux2/1 -> Terminator1/1
  Demux1/1 -> Terminator/1
  Product2/1 -> Sum3/1  "Ax . sin(dz)"
  Sum3/1 -> me2 . Le2/1
  me2 . Le2/1 -> Sum4/1
  Product1/1 -> Sum5/1  "Ax . sin(dy)"
  Product3/1 -> Sum3/2  "Ay . cos(dz)"
  Product/1 -> Sum5/2  "Az.cos(dy)"
  "Ie2 "/1 -> Sum2/2
  Sum4/1 -> switch1/1(in)
  Ie2/1 -> Sum4/2
  Sum2/1 -> switch/1(in)
  "me2 . Le2 "/1 -> Sum2/1
  Sum5/1 -> "me2 . Le2 "/1
  Ax/1 -> Product2/1, Product1/1
  Trigonometric Function/1 -> Product1/2
  Trigonometric Function1/1 -> Product/2
  Az/1 -> Product/1
  Trigonometric Function2/1 -> Product2/2
  Trigonometric Function3/1 -> Product3/2
  Ay/1 -> Product3/1
  R-dot/1 -> Ie2/1
  switch1/1(ou) -> TLz/1
  switch/1(ou) -> TLy/1

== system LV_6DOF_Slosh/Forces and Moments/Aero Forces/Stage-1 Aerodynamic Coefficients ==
  note: Aero Coefficients funct. of: Alpha, Beta, Mach#
  Incid : Inport
  Mach : Inport  Port=2
  Angle Conversion : aerolibconvert2/Angle Conversion  IU=rad  OU=deg
  Stage-1 Aero Coefficients : Subsystem
  Coeff : Outport  InitialOutput=0
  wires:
  Stage-1 Aero Coefficients/1(Coeff) -> Coeff/1
  Mach/1 -> Stage-1 Aero Coefficients/2(Mach)
  Angle Conversion/1 -> Stage-1 Aero Coefficients/1(albet)
  Incid/1 -> Angle Conversion/1

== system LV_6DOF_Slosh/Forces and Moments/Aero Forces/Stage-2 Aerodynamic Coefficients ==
  note: Aero Coefficients funct. of: Alpha, Beta, Mach#
  Incid : Inport
  Mach : Inport  Port=2
  Angle Conversion : aerolibconvert2/Angle Conversion  IU=rad  OU=deg
  Stage-2 Aero Coefficients : Subsystem
  Coeff : Outport  InitialOutput=0
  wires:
  Stage-2 Aero Coefficients/1(Coeff) -> Coeff/1
  Mach/1 -> Stage-2 Aero Coefficients/2(Mach)
  Angle Conversion/1 -> Stage-2 Aero Coefficients/1(albet)
  Incid/1 -> Angle Conversion/1

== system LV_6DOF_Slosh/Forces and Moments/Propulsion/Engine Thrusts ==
  note: Flow Rate
  note: Atmosph Pressure (psi)
  note: Thrust (lbf)
  note: Engine Thrusts Calculation
  Gain : Gain  Gain=2.012
  Gain1 : Gain  Gain=5.97
  Gain2 : Gain  Gain=32.174
  Ground : Ground
  Isp1 : Constant  Value=Isp1
  Isp2 : Constant  Value=Isp2
  Mux : Mux  Inputs=2
  Product1 : Product
  Product4 : Product
  Sum1 : Sum  Inputs=|+-
  Sum4 : Sum  Inputs=|+-
  Switch1 : Switch  Criteria=u2 > Threshold
  Switch2 : Switch  Criteria=u2 > Threshold
  Thrusts : ToWorkspace  VariableName=Teng  SampleTime=-1
  Thrust-1 : Outport
  Thrust-2 : Outport  Port=2
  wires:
  [s2_startup] -> Switch1/2
  [s1_shutdown] -> Switch2/2
  Mux/1 -> [Teng], Thrusts/1  "Thrust"
  Gain2/1 -> Product4/2, Product1/2
  Product4/1 -> Mux/1, Thrust-1/1
  Product1/1 -> Mux/2, Thrust-2/1
  Switch1/1 -> Product1/1  "ISP2"
  [Flow] -> Gain2/1
  Switch2/1 -> Product4/1  "ISP1"
  Gain1/1 -> Sum1/2
  Sum1/1 -> Switch1/1
  Gain/1 -> Sum4/2
  [atm] -> Gain/1, Gain1/1
  Isp1/1 -> Sum4/1
  Sum4/1 -> Switch2/3
  Ground/1 -> Switch2/1, Switch1/3
  Isp2/1 -> Sum1/1

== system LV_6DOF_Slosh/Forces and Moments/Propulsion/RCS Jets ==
  note: RCS Jet Forces (1-8)
  note: Fuel Counter
  note: Forces (X, Y, Z)
  note: Torques (X, Y, Z)
  note: RCS Forces and Torques
  RCS Jets : Inport
  Bottom +Y : Subsystem
  Bottom -Y : Subsystem
  Demux2 : Demux  Outputs=8
  Fcn : Fcn  Expr=(u(1)+u(2)+u(3)+u(4)+u(5)+u(6)+u(7)+u(8))/Isp
  Fuel : ToWorkspace  VariableName=Fuel  SampleTime=-1
  Integrator : Integrator
  Left +Z : Subsystem
  Left -Z : Subsystem
  Right +Z : Subsystem
  Right -Z : Subsystem
  Sum1 : Sum  Inputs=++++++++
  Sum4 : Sum  Inputs=++++++++
  Top +Y : Subsystem
  Top -Y : Subsystem
  Frcs : Outport
  Trcs : Outport  Port=2
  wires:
  Demux2/7 -> Left -Z/1(f(7))
  Right -Z/2(F8) -> Sum4/8
  Bottom -Y/2(F4) -> Sum4/4
  Bottom +Y/1(T2) -> Sum1/2
  Demux2/3 -> Top -Y/1(f(3))
  Demux2/2 -> Bottom +Y/1(f(2))
  Left -Z/2(F7) -> Sum4/7
  Top -Y/2(F3) -> Sum4/3
  Top +Y/2(F1) -> Sum4/1
  Top +Y/1(T1) -> Sum1/1
  Top -Y/1(T3) -> Sum1/3
  RCS Jets/1 -> Fcn/1, Demux2/1
  Demux2/8 -> Right -Z/1(f(8))
  Sum4/1 -> Frcs/1
  Demux2/5 -> Left +Z/1(f(5))
  Left +Z/2(F5) -> Sum4/5
  Bottom +Y/2(F2) -> Sum4/2
  Demux2/6 -> Right +Z/1(f(6))
  Demux2/1 -> Top +Y/1(f(1))
  Right +Z/2(F6) -> Sum4/6
  Right -Z/1(T8) -> Sum1/8
  Left -Z/1(T7) -> Sum1/7
  Bottom -Y/1(T4) -> Sum1/4
  Demux2/4 -> Bottom -Y/1(f(4))
  Integrator/1 -> Fuel/1
  Fcn/1 -> Integrator/1
  Left +Z/1(T5) -> Sum1/5
  Right +Z/1(T6) -> Sum1/6
  Sum1/1 -> Trcs/1

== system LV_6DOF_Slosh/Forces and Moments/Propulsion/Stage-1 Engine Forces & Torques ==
  note: Engine Forces and Torques
  note: Pitch Gimbal Deflections
  note: Yaw Gimbal Deflections
  note: Stage-1 Engines
  Thrst1 : Inport
  DY (rad) : Inport  Port=2
  DZ (rad) : Inport  Port=3
  Demux1 : Demux  Outputs=8
  Demux2 : Demux  Outputs=8
  Eng-1 : Subsystem
  Eng-2 : Subsystem
  Eng-3 : Subsystem
  Eng-4 : Subsystem
  Eng-5 : Subsystem
  Eng-6 : Subsystem
  Eng-7 : Subsystem
  Eng-8 : Subsystem
  Eng-9 Fixd : Subsystem
  Sum1 : Sum  Inputs=+++++++++
  Sum2 : Sum  Inputs=+++++++++
  Force : Outport  InitialOutput=0
  Torqu : Outport  Port=2  InitialOutput=0
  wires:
  DZ (rad)/1 -> Demux2/1
  Thrst1/1 -> Eng-4/1(Thrust), Eng-3/1(Thrust), Eng-2/1(Thrust), Eng-5/1(Thrust), Eng-8/1(Thrust), Eng-7/1(Thrust), Eng-6/1(Thrust), Eng-1/1(Thrust), Eng-9 Fixd/1(Thrust)
  Demux1/1 -> Eng-1/2(dy)
  Demux1/2 -> Eng-2/2(dy)
  Demux1/3 -> Eng-3/2(dy)
  Demux1/4 -> Eng-4/2(dy)
  Demux1/5 -> Eng-5/2(dy)
  Demux1/6 -> Eng-6/2(dy)
  Demux1/7 -> Eng-7/2(dy)
  Demux1/8 -> Eng-8/2(dy)
  Demux2/1 -> Eng-1/3(dz)
  Demux2/8 -> Eng-8/3(dz)
  Demux2/7 -> Eng-7/3(dz)
  Demux2/6 -> Eng-6/3(dz)
  Demux2/5 -> Eng-5/3(dz)
  Demux2/4 -> Eng-4/3(dz)
  Demux2/3 -> Eng-3/3(dz)
  Demux2/2 -> Eng-2/3(dz)
  Eng-1/2(M1) -> Sum2/1
  Eng-2/2(M2) -> Sum2/2
  Eng-3/2(M3) -> Sum2/3
  Eng-4/2(M4) -> Sum2/4
  Eng-8/2(M8) -> Sum2/8
  Eng-7/2(M7) -> Sum2/7
  Eng-6/2(M6) -> Sum2/6
  Eng-5/2(M5) -> Sum2/5
  Eng-1/1(F1) -> Sum1/1
  Eng-2/1(F2) -> Sum1/2
  Eng-3/1(F3) -> Sum1/3
  Eng-4/1(F4) -> Sum1/4
  Eng-8/1(F8) -> Sum1/8
  Eng-7/1(F7) -> Sum1/7
  Eng-6/1(F6) -> Sum1/6
  Eng-5/1(F5) -> Sum1/5
  DY (rad)/1 -> Demux1/1
  Sum1/1 -> Force/1
  Sum2/1 -> Torqu/1
  Eng-9 Fixd/1(F9) -> Sum1/9
  Eng-9 Fixd/2(M9) -> Sum2/9

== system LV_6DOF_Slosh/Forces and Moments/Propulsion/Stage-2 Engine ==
  note: Stage-2 Engine Force
  Thrst2 : Inport
  dy : Inport  Port=2
  dz : Inport  Port=3
  -1 : Gain  Gain=-1
  3x3 Cross Product : sharedutil/3x3 Cross Product  aMode=aMode
  Fx1 : Product  Inputs=3
  Fy1 : Product  Inputs=3
  Fz1 : Product
  Mux : Mux  Inputs=3
  Sum4 : Sum  Inputs=|++
  Thr*DThro : Product
  Throttle : TransferFcn  Numerator=[5]  Denominator="[1  5]"
  cos(dy) : Trigonometry  Operator=cos
  cos(dz) : Trigonometry  Operator=cos
  sin(dy) : Trigonometry
  sin(dz) : Trigonometry
  F10 : Outport  InitialOutput=0
  M10 : Outport  Port=2  InitialOutput=0
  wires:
  Sum4/1 -> Fy1/1, Fx1/1, -1/1
  3x3 Cross Product/1 -> M10/1
  [lg10] -> 3x3 Cross Product/1
  cos(dy)/1 -> Fy1/2, Fx1/2
  -1/1 -> Fz1/1
  Fy1/1 -> Mux/2
  Fz1/1 -> Mux/3
  Fx1/1 -> Mux/1
  Mux/1 -> F10/1, 3x3 Cross Product/2
  cos(dz)/1 -> Fx1/3
  sin(dz)/1 -> Fy1/3
  sin(dy)/1 -> Fz1/2
  dy/1 -> cos(dy)/1, sin(dy)/1
  dz/1 -> cos(dz)/1, sin(dz)/1
  Thr*DThro/1 -> Sum4/1
  Thrst2/1 -> Sum4/2, Thr*DThro/2
  Throttle/1 -> Thr*DThro/1
  [DThro] -> Throttle/1

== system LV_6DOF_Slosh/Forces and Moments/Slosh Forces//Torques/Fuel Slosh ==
  note: Slosh Mass
  note: Pendulum Angle (rad)
  note: Non-Linear Fuel Pendulum Model
  note: Vehicle Acceleration Ax, Ay, Az at Tank
  note: Slosh Mass Position Velocity, Acceleration Relative to Tank Center
  note: Angular Rate (r/s)
  note: Damping Coeff.
  note: Pendul Length
  note: String Extension
  note: Slosh Forces on Vehicle: Fy, Fz
  Axyz : Inport
  "  Xs" : ToWorkspace  VariableName=Xsb  SampleTime=-1
  "  theta" : ToWorkspace  VariableName=thetb  SampleTime=-1
  " Fv" : ToWorkspace  VariableName=Fvb  SampleTime=-1
  " Xsd " : ToWorkspace  VariableName=Xsdb  SampleTime=-1
  " Xsdd " : ToWorkspace  VariableName=Xsddb  SampleTime=-1
  " delta" : ToWorkspace  VariableName=delb  SampleTime=-1
  " u1" : ToWorkspace  VariableName=u1b  SampleTime=-1
  " u2" : ToWorkspace  VariableName=u2b  SampleTime=-1
  Demux1 : Demux  Outputs="[3,  3]"
  Demux2 : Demux  Outputs="[3,  3]"
  Fyz : Selector  InputPortWidth=3  IndexOptions=Index vector (dialog)  Indices=[2,3]  OutputSizes=1
  Integrator : Integrator  InitialCondition="[0,0,velpnd,  -0.5*cosd(thpnd), 0.5*sind(thpnd), 0]"
  MATLAB Function : MATLAB Function  TreatAsAtomicUnit=on
  Memory : Memory  InheritSampleTime=on
  "Ms_fuel " : Lookup  InputValues=Mvsls  Table=Msfue
  R_fuel : Lookup  InputValues=Mvsls  Table=Rfuel
  Terminator : Terminator
  "Wsl " : ToWorkspace  VariableName=Wslb  SampleTime=-1
  Zeta_fuel : Lookup  InputValues=Mvsls  Table=Ztfue
  Ffuel : Outport
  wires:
  [mass] -> R_fuel/1, Zeta_fuel/1, "Ms_fuel "/1
  MATLAB Function/7(theta) -> "  theta"/1
  Demux2/1 -> " Xsdd "/1
  Demux1/2 -> "  Xs"/1
  Demux1/1 -> " Xsd "/1
  R_fuel/1 -> MATLAB Function/4(Rsl)
  MATLAB Function/6(Wsl) -> "Wsl "/1
  MATLAB Function/5(delta) -> " delta"/1
  MATLAB Function/3(u2) -> " u2"/1
  MATLAB Function/2(u1) -> " u1"/1
  Integrator/1 -> Demux1/1, MATLAB Function/1(x)  "x"
  MATLAB Function/1(xdot) -> Integrator/1, Demux2/1
  Demux2/2 -> Terminator/1
  "Ms_fuel "/1 -> MATLAB Function/3(Msl)
  Zeta_fuel/1 -> MATLAB Function/5(Zeta)
  Memory/1 -> MATLAB Function/2(Acc)
  Fyz/1 -> [Fsfuel], " Fv"/1
  MATLAB Function/4(Fv) -> Ffuel/1, Fyz/1
  Axyz/1 -> Memory/1

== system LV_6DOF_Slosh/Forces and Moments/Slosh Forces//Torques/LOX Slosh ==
  note: Slosh Mass
  note: Pendulum Angle (rad)
  note: Non-Linear LOX Pendulum Model
  note: Vehicle Acceleration Ax, Ay, Az at Tank
  note: Slosh Mass Position Velocity, Acceleration Relative to Tank Center
  note: Slosh Forces on Vehicle: Fy, Fz
  note: String Extension
  note: Angular Rate (r/s)
  note: Damping Coeff.
  note: Pendul Length
  Axyz : Inport
  "  Xs" : ToWorkspace  VariableName=Xsa  SampleTime=-1
  "  theta" : ToWorkspace  VariableName=theta  SampleTime=-1
  " Fv" : ToWorkspace  VariableName=Fva  SampleTime=-1
  " Xsd" : ToWorkspace  VariableName=Xsda  SampleTime=-1
  " Xsdd" : ToWorkspace  VariableName=Xsdda  SampleTime=-1
  " delta" : ToWorkspace  VariableName=dela  SampleTime=-1
  " u1" : ToWorkspace  VariableName=u1a  SampleTime=-1
  " u2" : ToWorkspace  VariableName=u2a  SampleTime=-1
  Demux1 : Demux  Outputs="[3,  3]"
  Demux2 : Demux  Outputs="[3,  3]"
  Fyz : Selector  InputPortWidth=3  IndexOptions=Index vector (dialog)  Indices=[2,3]  OutputSizes=1
  Integrator : Integrator  InitialCondition="[0,0,velpnd,  -0.5*cosd(thpnd), 0, -0.5*sind(thpnd)]"
  MATLAB Function : MATLAB Function  TreatAsAtomicUnit=on
  Memory : Memory  InheritSampleTime=on
  "Ms_lox " : Lookup  InputValues=Mvsls  Table=Mslox
  R_lox : Lookup  InputValues=Mvsls  Table=Rlox
  Terminator : Terminator
  Wsl : ToWorkspace  VariableName=Wsla  SampleTime=-1
  Zeta_lox : Lookup  InputValues=Mvsls  Table=Ztlox
  Flox : Outport
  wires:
  [mass] -> R_lox/1, Zeta_lox/1, "Ms_lox "/1
  MATLAB Function/7(theta) -> "  theta"/1
  Demux2/1 -> " Xsdd"/1
  Demux1/2 -> "  Xs"/1
  Demux1/1 -> " Xsd"/1
  R_lox/1 -> MATLAB Function/4(Rsl)
  MATLAB Function/6(Wsl) -> Wsl/1
  MATLAB Function/5(delta) -> " delta"/1
  MATLAB Function/3(u2) -> " u2"/1
  MATLAB Function/2(u1) -> " u1"/1
  Integrator/1 -> MATLAB Function/1(x), Demux1/1  "x"
  MATLAB Function/1(xdot) -> Integrator/1, Demux2/1
  Demux2/2 -> Terminator/1
  MATLAB Function/4(Fv) -> Flox/1, Fyz/1
  "Ms_lox "/1 -> MATLAB Function/3(Msl)
  Zeta_lox/1 -> MATLAB Function/5(Zeta)
  Memory/1 -> MATLAB Function/2(Acc)
  Fyz/1 -> [Fslox], " Fv"/1
  Axyz/1 -> Memory/1

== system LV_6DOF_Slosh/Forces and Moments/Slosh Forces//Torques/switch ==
  in : Inport
  Ground : Ground
  Slosh Switch : Constant  Value=Islosh
  Switch : Switch  Criteria=u2 > Threshold  Threshold=0.5
  ou : Outport
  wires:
  Slosh Switch/1 -> Switch/2
  in/1 -> Switch/1
  Switch/1 -> ou/1
  Ground/1 -> Switch/3

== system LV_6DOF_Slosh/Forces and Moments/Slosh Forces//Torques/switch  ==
  in : Inport
  Ground : Ground
  Slosh Switch : Constant  Value=Islosh
  Switch : Switch  Criteria=u2 > Threshold  Threshold=0.5
  ou : Outport
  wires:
  Slosh Switch/1 -> Switch/2
  in/1 -> Switch/1
  Switch/1 -> ou/1
  Ground/1 -> Switch/3

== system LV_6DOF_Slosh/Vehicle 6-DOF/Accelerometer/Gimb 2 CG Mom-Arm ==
  note: Gimbal-CG Moment Arm (ft)
  Sum1 : Sum  Inputs=|+-
  Sum3 : Sum  Inputs=|+-
  Switch1 : Switch  Criteria=u2 > Threshold
  Switch2 : Switch  Criteria=u2 > Threshold
  Switch3 : Switch  Criteria=u2 > Threshold
  Xgimb1 : Constant  Value=[Xgmb1,0,0]
  Xgimb2 : Constant  Value=[Xgmb2, 0, 0]
  Lg : Outport
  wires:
  Xgimb1/1 -> Switch1/3
  Xgimb2/1 -> Switch2/1
  [s2_startup] -> Switch2/2
  [stage_sep] -> Switch1/2
  Switch1/1 -> Sum3/1
  Switch2/1 -> Sum1/1
  Sum1/1 -> Switch3/1
  Sum3/1 -> Switch3/3
  Switch3/1 -> Lg/1
  [s2_startup] -> Switch3/2
  [CG] -> Sum1/2, Switch2/3, Switch1/1, Sum3/2

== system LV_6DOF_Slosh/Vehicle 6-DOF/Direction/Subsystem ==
  Vx : Inport
  Vy : Inport  Port=2
  Product : Product
  Product1 : Product
  Sqrt : Sqrt
  Sum : Sum  Inputs=|++
  Vxy : Outport
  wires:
  Sqrt/1 -> Vxy/1
  Vy/1 -> Product1/2, Product1/1
  Sum/1 -> Sqrt/1
  Product1/1 -> Sum/2
  Product/1 -> Sum/1
  Vx/1 -> Product/2, Product/1

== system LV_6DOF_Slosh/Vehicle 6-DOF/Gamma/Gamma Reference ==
  Demux : Demux  Tag=STV Demux  Outputs=1
  FromWs : FromWorkspace  Tag=STV FromWs  VariableName=tuvar  SampleTime=0
  Gama_cmd : Outport  Tag=STV Outport
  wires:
  FromWs/1 -> Demux/1
  Demux/1 -> Gama_cmd/1

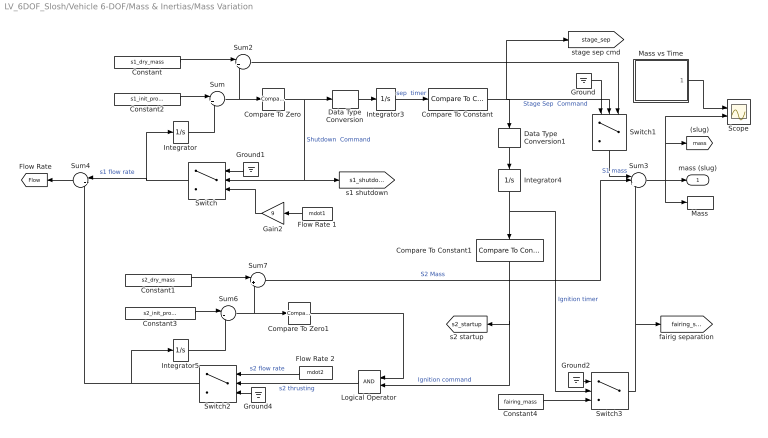
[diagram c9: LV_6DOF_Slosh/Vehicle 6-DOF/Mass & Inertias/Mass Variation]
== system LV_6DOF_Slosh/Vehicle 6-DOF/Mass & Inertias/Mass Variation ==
  Compare To Constant : simulink/Logic and Bit Operations/Compare To Constant  relop=>=  const=pre_sep_wait  OutDataTypeStr=uint8
  Compare To Constant1 : simulink/Logic and Bit Operations/Compare To Constant  relop=>=  const=post_sep_wait  OutDataTypeStr=boolean
  Compare To Zero : simulink/Logic and Bit Operations/Compare To Zero  relop=<=  OutDataTypeStr=uint8
  Compare To Zero1 : simulink/Logic and Bit Operations/Compare To Zero  relop=>  OutDataTypeStr=boolean
  Constant : Constant  Value=s1_dry_mass
  Constant1 : Constant  Value=s2_dry_mass
  Constant2 : Constant  Value=s1_init_prop_mass
  Constant3 : Constant  Value=s2_init_prop_mass
  Constant4 : Constant  Value=fairing_mass
  Data Type Conversion : DataTypeConversion  OutDataTypeStr=double
  Data Type Conversion1 : DataTypeConversion  OutDataTypeStr=double
  Flow Rate 1 : Constant  Value=mdot1
  Flow Rate 2 : Constant  Value=mdot2
  Gain2 : Gain  Gain=9
  Ground{,1..2,4} (4 alike) : Ground
  Integrator{,3..5} (4 alike) : Integrator
  Logical Operator : Logic  AllPortsSameDT=off  OutDataTypeStr=boolean
  Mass : ToWorkspace  VariableName=mass  SampleTime=-1
  Mass vs Time : Subsystem  Tag=STV Subsys  LoadFcn=sigbuilder_block('load');  StartFcn=sigbuilder_block('start');  StopFcn=sigbuilder_block('stop');  ClipboardFcn=sigbuilder_block('clipboard');  mask(Sigbuilder block){tuvar=[0:10]}
      mask help: Sigbuilder GUI
      mask init:
      | if ~strcmp(get_param(bdroot(gcbh),'SimulationStatus'),'stopped') tuvar = sigbuilder_block('maskInit'); end
  Scope : Scope  NumInputPorts=2
  Sum : Sum  Inputs=|+-
  Sum2 : Sum  Inputs=|++
  Sum3 : Sum  Inputs=|+++
  Sum4 : Sum  Inputs=|++
  Sum6 : Sum  Inputs=|+-
  Sum7 : Sum  Inputs=|++
  Switch : Switch  Criteria=u2 > Threshold
  Switch1 : Switch  Criteria=u2 > Threshold
  Switch2 : Switch  Criteria=u2 > Threshold
  Switch3 : Switch  Criteria=u2 > Threshold  Threshold=stage_to_fairing_sep_time
  mass (slug) : Outport
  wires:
  Ground/1 -> Switch1/1
  Switch3/1 -> Sum3/3, [fairing_sep]
  Ground2/1 -> Switch3/1
  Constant4/1 -> Switch3/3
  Data Type Conversion/1 -> Integrator3/1
  Data Type Conversion1/1 -> Integrator4/1
  Constant1/1 -> Sum7/1
  Sum4/1 -> [Flow]
  Compare To Constant1/1 -> Logical Operator/2, [s2_startup]  "Ignition command"
  Compare To Zero1/1 -> Logical Operator/1
  Sum7/1 -> Sum3/2  "S2 Mass"
  Sum6/1 -> Compare To Zero1/1, Sum7/2
  Constant3/1 -> Sum6/1
  Integrator5/1 -> Sum6/2
  Switch2/1 -> Sum4/2, Integrator5/1
  Ground4/1 -> Switch2/3
  Flow Rate 2/1 -> Switch2/1  "s2 flow rate"
  Logical Operator/1 -> Switch2/2  "s2 thrusting"
  Integrator4/1 -> Compare To Constant1/1, Switch3/2  "Ignition timer"
  Switch1/1 -> Sum3/1  "S1 mass"
  Compare To Constant/1 -> Switch1/2, [stage_sep], Data Type Conversion1/1  "Stage Sep  Command"
  Sum2/1 -> Switch1/3
  Integrator3/1 -> Compare To Constant/1  "sep  timer"
  Switch/1 -> Integrator/1, Sum4/1  "s1 flow rate"
  Gain2/1 -> Switch/3
  Ground1/1 -> Switch/1
  Compare To Zero/1 -> Data Type Conversion/1, [s1_shutdown], Switch/2  "Shutdown  Command"
  Sum/1 -> Compare To Zero/1, Sum2/2
  Integrator/1 -> Sum/2
  Constant2/1 -> Sum/1
  Constant/1 -> Sum2/1
  Flow Rate 1/1 -> Gain2/1
  Sum3/1 -> Scope/2, [mass], Mass/1, mass (slug)/1
  Mass vs Time/1(Mass (slg)) -> Scope/1

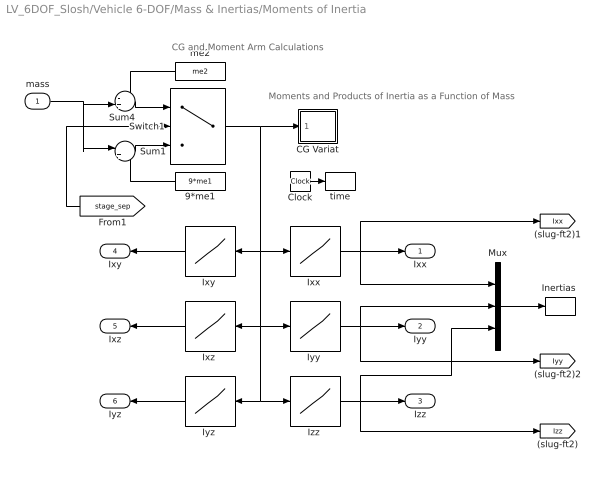
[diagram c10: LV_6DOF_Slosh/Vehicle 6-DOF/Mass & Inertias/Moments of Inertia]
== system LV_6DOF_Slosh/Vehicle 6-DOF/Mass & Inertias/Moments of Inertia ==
  note: Moments and Products of Inertia as a Function of Mass
  note: CG and Moment Arm Calculations
  mass : Inport
  9*me1 : Constant  Value=9*me1
  CG Variat : Subsystem
  Clock : Clock
  "Inertias " : ToWorkspace  VariableName=MOI  SampleTime=-1
  "Ixx " : Lookup  InputValues=msspr  Table=Ixxpr
  "Ixy " : Lookup  InputValues=msspr  Table=Ixypr
  "Ixz " : Lookup  InputValues=msspr  Table=Ixzpr
  "Iyy " : Lookup  InputValues=msspr  Table=Iyypr
  "Iyz " : Lookup  InputValues=msspr  Table=Iyzpr
  "Izz " : Lookup  InputValues=msspr  Table=Izzpr
  Mux : Mux  Inputs=3
  Sum1 : Sum  Inputs=|+-
  Sum4 : Sum  Inputs=-+|
  Switch1 : Switch  Criteria=u2 > Threshold
  me2 : Constant  Value=me2
  time : ToWorkspace  VariableName=time  SampleTime=-1
  Ixx : Outport
  Iyy : Outport  Port=2
  Izz : Outport  Port=3
  Ixy : Outport  Port=4
  Ixz : Outport  Port=5
  Iyz : Outport  Port=6
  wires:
  Switch1/1 -> CG Variat/1(m), "Iyz "/1, "Izz "/1, "Ixz "/1, "Iyy "/1, "Ixy "/1, "Ixx "/1
  "Ixx "/1 -> [Ixx], Ixx/1, Mux/1
  "Iyy "/1 -> [Iyy], Iyy/1, Mux/2
  "Izz "/1 -> [Izz], Izz/1, Mux/3
  "Ixy "/1 -> Ixy/1
  "Ixz "/1 -> Ixz/1
  "Iyz "/1 -> Iyz/1
  Mux/1 -> "Inertias "/1
  [stage_sep] -> Switch1/2
  Sum4/1 -> Switch1/1
  mass/1 -> Sum1/1, Sum4/2
  Sum1/1 -> Switch1/3
  9*me1/1 -> Sum1/2
  me2/1 -> Sum4/1
  Clock/1 -> time/1

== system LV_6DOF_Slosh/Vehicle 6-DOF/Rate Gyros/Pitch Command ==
  Demux : Demux  Tag=STV Demux  Outputs=1
  FromWs : FromWorkspace  Tag=STV FromWs  VariableName=tuvar  SampleTime=0
  Theta_cmd : Outport  Tag=STV Outport
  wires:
  FromWs/1 -> Demux/1
  Demux/1 -> Theta_cmd/1

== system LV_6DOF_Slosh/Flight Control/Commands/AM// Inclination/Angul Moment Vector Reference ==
  note: Angular Momentum Reference
  1-D Lookup Table : Lookup_n-D  NumberOfTableDimensions=1  BreakpointsForDimension1=timi2  Table=JJ1  InternalRulePriority=Speed  RndMeth=Simplest
  1-D Lookup Table1 : Lookup_n-D  NumberOfTableDimensions=1  BreakpointsForDimension1=timi2  Table=JJ2  InternalRulePriority=Speed  RndMeth=Simplest
  1-D Lookup Table2 : Lookup_n-D  NumberOfTableDimensions=1  BreakpointsForDimension1=timi2  Table=JJ3  InternalRulePriority=Speed  RndMeth=Simplest
  Clock : Clock
  Mux1 : Mux  Inputs=3
  J3 : Outport
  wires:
  1-D Lookup Table1/1 -> Mux1/2
  Clock/1 -> 1-D Lookup Table/1, 1-D Lookup Table1/1, 1-D Lookup Table2/1
  1-D Lookup Table2/1 -> Mux1/3
  Mux1/1 -> J3/1
  1-D Lookup Table/1 -> Mux1/1

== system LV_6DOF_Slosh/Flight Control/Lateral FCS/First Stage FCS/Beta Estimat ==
  note: Qbar*Sref*Cyb*beta
  note: Beta Estimator
  r : Inport
  dz : Inport  Port=2
  1/9 : Gain  Gain=1/9
  3 : Gain  Gain=15
  Cybeta : Lookup  InputValues=Vrelgn1  Table=Cza1
  Demux : Demux  Outputs=8
  Mass : Product
  Ny Washout : TransferFcn  Numerator="[1  0]"  Denominator="[0.015  1]"
  Product : Product  Inputs=4
  Qbar : Lookup  InputValues=Vrelgn1  Table=Qbar1
  Selector : Selector  InputPortWidth=3  IndexOptions=Index vector (dialog)  Indices=[2]  OutputSizes=1
  Selector1 : Selector  InputPortWidth=2  IndexOptions=Index vector (dialog)  Indices=[1]  OutputSizes=1
  Slosh-Notch : Subsystem
  Sref : Constant  Value=Sref
  Sum : Sum  Inputs=-+|
  Sum of Elements : Sum  Inputs=++++++++
  Sum2 : Sum  Inputs=-+-
  Thrust*dz : Product
  d2r : Gain  Gain=d2r
  betest : Outport
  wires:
  Sum2/1 -> Slosh-Notch/1(In)
  r/1 -> Ny Washout/1
  Product/1 -> Sum2/3
  Mass/1 -> Sum2/1
  d2r/1 -> betest/1
  Sum/1 -> Mass/2
  [mass] -> Mass/1
  [V0] -> Qbar/1, Cybeta/1
  Qbar/1 -> Product/4
  Sref/1 -> Product/2
  Cybeta/1 -> Product/3
  [Axlrm] -> Selector/1  "(ft/sec^2)"
  Selector/1 -> Sum/2  "Ydd"
  1/9/1 -> Thrust*dz/1
  Selector1/1 -> 1/9/1
  Sum of Elements/1 -> Thrust*dz/2
  Demux/5 -> Sum of Elements/5
  [Teng] -> Selector1/1  "(lbf)"
  Demux/4 -> Sum of Elements/4
  Demux/1 -> Sum of Elements/1
  Demux/2 -> Sum of Elements/2
  Thrust*dz/1 -> Sum2/2  "Fy"
  dz/1 -> Demux/1  "(rad)"
  Demux/6 -> Sum of Elements/6
  Demux/8 -> Sum of Elements/8
  Demux/7 -> Sum of Elements/7
  Demux/3 -> Sum of Elements/3
  Ny Washout/1 -> 3/1
  3/1 -> Sum/1
  Slosh-Notch/1(Out) -> Product/1, d2r/1  "beta (deg)"

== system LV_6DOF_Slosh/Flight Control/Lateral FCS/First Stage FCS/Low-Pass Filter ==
  note: Variable Low Pass Filter
  u : Inport
  2.zet.w : Subsystem
  Sum2 : Sum  Inputs=|+-
  Sum3 : Sum  Inputs=-+|
  int1 : Integrator
  int2 : Integrator
  "w^2 " : Subsystem
  y : Outport
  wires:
  Sum3/1 -> "w^2 "/1(in)
  int1/1 -> 2.zet.w/1(in), int2/1
  Sum2/1 -> int1/1
  "w^2 "/1(ou) -> Sum2/1
  2.zet.w/1(ou) -> Sum2/2
  int2/1 -> Sum3/1, y/1
  u/1 -> Sum3/2
